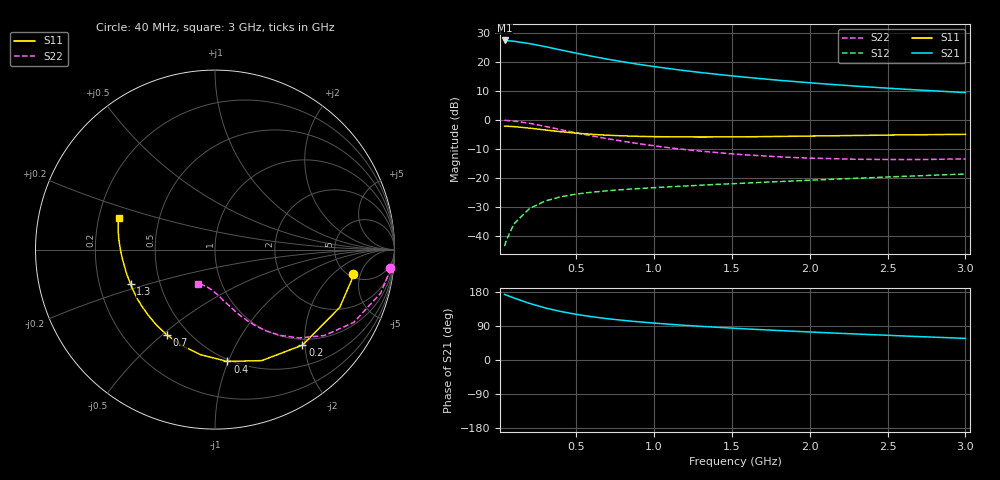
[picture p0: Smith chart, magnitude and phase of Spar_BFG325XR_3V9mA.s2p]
! Filename: 39BFG325XR.s2p
! Title: BFG325XR,RN20042071,Lot:TT3899C,B:Y13641,Sl.:1
! Bias: VCE=2.999V; IC=8.923mA;
! Company: NXP Semiconductors NL
! User: Q&R DSC-N
! Measure time: 29 Mar 2004 / 13:39:28
#  MHz  S  MA  R 50
! Freq  S11  S21  S12  S22  :
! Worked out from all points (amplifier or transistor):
!   32 points, 40 MHz to 3 GHz, reference 50 ohm
!   highest |S21| = 27.3 dB at 40 MHz (marker M1)
!   |S21| within 3 dB of that: start of sweep to 377.7 MHz
!   unconditionally stable (mu >= 1): 2.294 GHz to end of sweep
!   at 400 MHz: K = 0.32, MSG = 25.2 dB, |S12| = -26.4 dB
!   at 1.5 GHz: K = 0.85, MSG = 18.5 dB, |S12| = -21.9 dB
!   at 3 GHz: K = 1.04, MAG = 12.7 dB, |S12| = -18.6 dB
!   S11 on the Smith chart (normalised r, x): 40 MHz: 5.41, -3.79; 200 MHz: 0.88, -1.95; 400 MHz: 0.48, -0.99; 700 MHz: 0.38, -0.52; 1.3 GHz: 0.34, -0.18; 3 GHz: 0.29, +0.15
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40  0.781 -10.1  23.11 173.1  0.006784 85.0  0.9823 -5.9
50  0.7798 -12.6  23 171.4  0.008447 83.5  0.9796 -7.4
100  0.766 -24.9  22.38 163.6  0.01642 77.4  0.9546 -14.7
200  0.7214 -47.6  20.42 149.3  0.03011 66.8  0.8732 -27.7
300  0.6711 -67.2  18.11 137.5  0.04038 58.7  0.7749 -38.1
400  0.6267 -83.7  15.89 128.1  0.04776 52.8  0.68 -46.4
500  0.5914 -97.7  13.97 120.5  0.05322 48.8  0.5988 -52.9
600  0.5647 -109.5  12.38 114.2  0.05731 46.0  0.5315 -58.1
700  0.5455 -119.5  11.04 109.0  0.06061 44.2  0.4753 -62.4
800  0.5318 -128.1  9.933 104.7  0.06358 43.0  0.4289 -66.0
900  0.5215 -135.6  9.013 100.8  0.0661 42.3  0.391 -69.3
1000  0.5152 -142.2  8.23 97.4  0.06855 41.8  0.3593 -72.1
1100  0.5122 -147.9  7.57 94.3  0.07096 41.6  0.3314 -74.8
1200  0.5094 -153.0  6.997 91.5  0.0732 41.6  0.3089 -77.5
1300  0.508 -157.7  6.505 88.8  0.07552 41.7  0.2908 -80.1
1500  0.511 -165.6  5.696 84.2  0.08012 42.2  0.261 -84.8
1600  0.5126 -169.1  5.366 81.9  0.08232 42.3  0.2495 -87.3
1800  0.5198 -175.2  4.79 77.8  0.08707 42.9  0.2325 -91.9
2100  0.5314 177.3  4.136 72.1  0.0943 43.5  0.2173 -98.8
2400  0.5436 171.3  3.643 66.8  0.1018 44.1  0.2099 -105.2
2600  0.5521 167.9  3.373 63.5  0.1072 44.4  0.2083 -109.0
3000  0.5639 161.9  2.948 57.0  0.1176 44.2  0.2135 -116.2
